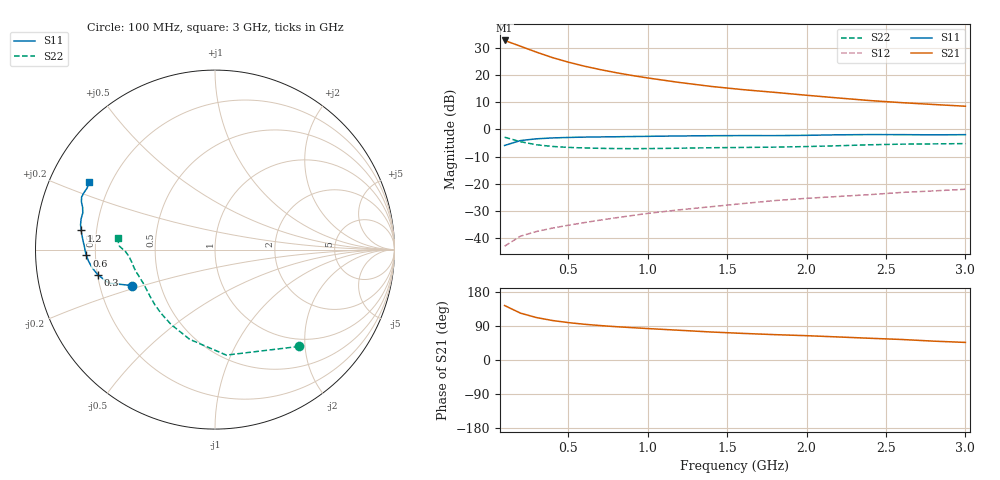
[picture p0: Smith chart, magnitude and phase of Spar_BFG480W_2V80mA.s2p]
! Filename: 280BFG480.001
! Title: BFG480W
! Bias: Vce=2V; Ic=80mA
! Company: NXP Semiconductors NL
! User: Quality&Reliability T&D
! Measure time: 10 Nov 1999 / 11:54:36
#  MHz  S  MA  R 50
! Freq  S11  S21  S12  S22  :
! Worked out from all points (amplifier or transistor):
!   20 points, 100 MHz to 3 GHz, reference 50 ohm
!   highest |S21| = 32.6 dB at 100 MHz (marker M1)
!   |S21| within 3 dB of that: start of sweep to 240.7 MHz
!   unconditionally stable (mu >= 1): 707.9 MHz to end of sweep
!   at 400 MHz: K = 0.81, MSG = 31.3 dB, |S12| = -36.3 dB
!   at 1.2 GHz: K = 1.09, MAG = 21.6 dB, |S12| = -29.6 dB
!   at 3 GHz: K = 1.10, MAG = 13.3 dB, |S12| = -22.0 dB
!   S11 on the Smith chart (normalised r, x): 100 MHz: 0.34, -0.18; 300 MHz: 0.20, -0.10; 600 MHz: 0.16, -0.02; 1.2 GHz: 0.14, +0.07; 3 GHz: 0.12, +0.25
100  0.5046 -156.6  42.64 143.7  0.007154 67.4  0.7149 -49.0
200  0.6209 -162.5  33.41 123.6  0.01093 57.8  0.5913 -83.9
300  0.668 -167.9  26.04 112.0  0.01329 56.7  0.5193 -105.8
400  0.6931 -171.8  20.71 104.3  0.01533 58.2  0.4838 -120.3
500  0.7075 -174.8  17.08 98.7  0.01731 60.2  0.465 -130.4
600  0.7176 -177.4  14.43 94.4  0.01935 62.0  0.4541 -137.8
700  0.7238 -179.6  12.48 90.9  0.02148 64.1  0.4468 -143.4
800  0.7285 178.4  10.95 87.9  0.02372 65.9  0.4425 -148.0
900  0.7354 176.6  9.728 85.4  0.02605 67.6  0.441 -151.9
1000  0.7417 174.8  8.755 83.0  0.02855 68.6  0.442 -155.4
1200  0.7534 171.9  7.225 78.4  0.03325 70.2  0.4493 -160.9
1400  0.7616 169.5  6.11 73.9  0.0379 71.2  0.4583 -165.0
1600  0.7654 167.1  5.335 70.2  0.04331 71.9  0.4635 -168.3
1800  0.7645 164.5  4.756 66.9  0.04913 72.4  0.4701 -171.8
2000  0.774 162.3  4.208 64.2  0.05403 72.9  0.4814 -175.6
2200  0.7912 160.2  3.752 60.8  0.05843 73.0  0.4986 -178.7
2400  0.7988 158.5  3.361 57.3  0.06317 72.5  0.519 179.2
2600  0.7966 156.7  3.077 54.1  0.06932 71.8  0.5332 177.9
2800  0.7906 154.4  2.849 49.7  0.07394 70.4  0.5391 176.1
3000  0.7961 151.7  2.647 46.4  0.07921 69.6  0.5454 173.3
